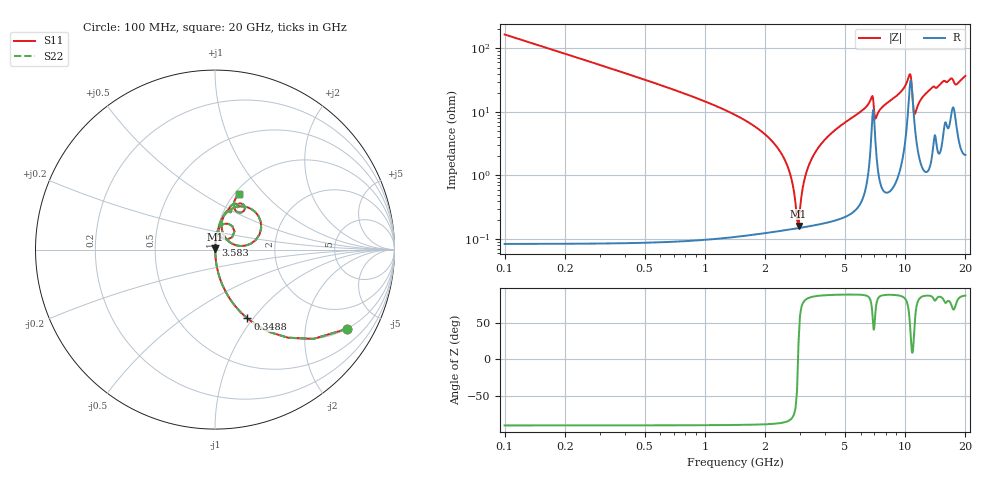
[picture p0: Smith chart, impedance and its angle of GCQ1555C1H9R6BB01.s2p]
!Murata Part Number: GCQ1555C1H9R6BB01
!These Parameters are Measured in Series Mode Connection
!Data Generated on Jan 08, 2026
!  o--ll--o
!Port1  Port2
!  o------o
!Operation Temp=25[degC], DC Bias Voltage=0[V]
!Freq. Start=100[MHz] Stop=20[GHz] 401[Steps]
# Hz S RI R 50
!Freq.(Hz) S11(Real) S11(Imag) S21(Real) S21(Imag) S12(Real) S12(Imag) S22(Real) S22(Imag)
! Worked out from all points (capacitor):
!   401 points, 100 MHz to 20 GHz, reference 50 ohm
!   read as one part in series: C = 9.6 pF near 199.5 MHz
!   lowest |Z| = 160 mohm at 2.936 GHz (marker M1)
!   series resonance near 2.92 GHz, so ESL is about 310 pH
!   S11 on the Smith chart (normalised r, x): 100 MHz: 1.00, -3.31; 348.8 MHz: 1.00, -0.94; 3.583 GHz: 1.00, +0.05; 20 GHz: 1.04, +0.74
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1e8  0.7327 -0.4423  0.2673 0.4423  0.2673 0.4423  0.7327 -0.4423
3.4875e8  0.1805 -0.3837  0.8195 0.3837  0.8195 0.3837  0.1805 -0.3837
9.955e8  0.0221 -0.1439  0.9779 0.1439  0.9779 0.1439  0.0221 -0.1439
2.33875e9  0.00197 -0.0255  0.998 0.0255  0.998 0.0255  0.00197 -0.0255
2.63725e9  0.00154 -0.0117  0.9985 0.0117  0.9985 0.0117  0.00154 -0.0117
2.83625e9  0.00146 -0.00334  0.9985 0.00334  0.9985 0.00334  0.00146 -0.00334
2.93575e9  0.00148 0.000606  0.9985 -0.000606  0.9985 -0.000606  0.00148 0.000606
3.1845e9  0.00164 0.00996  0.9984 -0.00996  0.9984 -0.00996  0.00164 0.00996
3.43325e9  0.00196 0.0187  0.998 -0.0187  0.998 -0.0187  0.00196 0.0187
3.5825e9  0.00222 0.0238  0.9978 -0.0238  0.9978 -0.0238  0.00222 0.0238
4.478e9  0.00463 0.0517  0.9954 -0.0517  0.9954 -0.0517  0.00463 0.0517
6.7665e9  0.0581 0.1445  0.9419 -0.1445  0.9419 -0.1445  0.0581 0.1445
7.1645e9  0.029 0.074  0.971 -0.074  0.971 -0.074  0.029 0.074
1.005e10  0.0942 0.228  0.9058 -0.228  0.9058 -0.228  0.0942 0.228
1.059725e10  0.2547 0.1565  0.7453 -0.1565  0.7453 -0.1565  0.2547 0.1565
1.0846e10  0.1692 0.022  0.8308 -0.022  0.8308 -0.022  0.1692 0.022
1.11445e10  0.0647 0.0576  0.9353 -0.0576  0.9353 -0.0576  0.0647 0.0576
1.199025e10  0.0377 0.1481  0.9623 -0.1481  0.9623 -0.1481  0.0377 0.1481
1.338325e10  0.0616 0.2103  0.9384 -0.2103  0.9384 -0.2103  0.0616 0.2103
1.67165e10  0.1386 0.2574  0.8614 -0.2574  0.8614 -0.2574  0.1386 0.2574
1.79105e10  0.1186 0.2137  0.8814 -0.2137  0.8814 -0.2137  0.1186 0.2137
2e10  0.1332 0.3125  0.8668 -0.3125  0.8668 -0.3125  0.1332 0.3125
